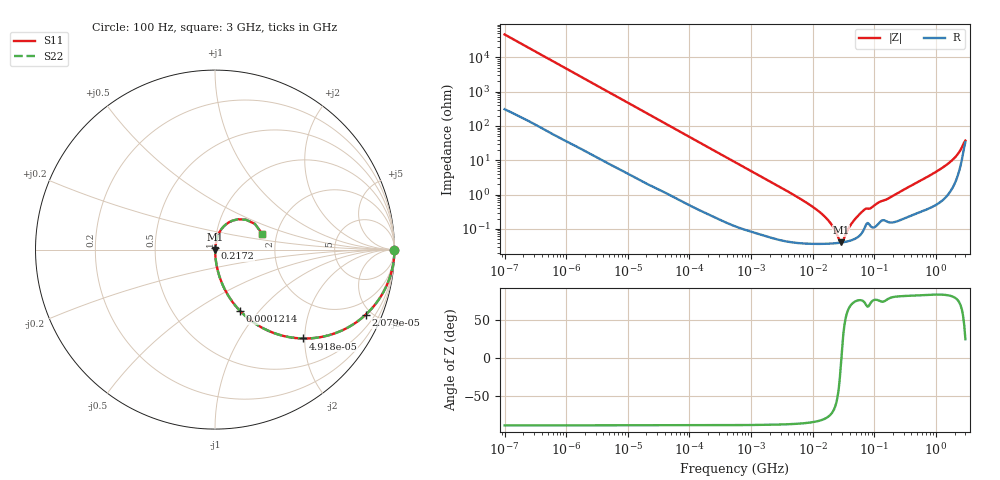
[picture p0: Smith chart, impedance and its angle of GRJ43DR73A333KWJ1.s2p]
!Murata Part Number: GRJ43DR73A333KWJ1
!These Parameters are Measured in Series Mode Connection
!Data Generated on Jun 19, 2026
!  o--ll--o
!Port1  Port2
!  o------o
!Operation Temp=25[degC], DC Bias Voltage=0[V]
!Freq. Start=100[Hz] Stop=3[GHz] 401[Steps]
# Hz S RI R 50
!Freq.(Hz) S11(Real) S11(Imag) S21(Real) S21(Imag) S12(Real) S12(Imag) S22(Real) S22(Imag)
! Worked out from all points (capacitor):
!   401 points, 100 Hz to 3 GHz, reference 50 ohm
!   read as one part in series: C = 34.1 nF near 109 Hz
!   lowest |Z| = 40.1 mohm at 28.73 MHz (marker M1)
!   series resonance near 29.17 MHz, so ESL is about 870 pH
!   S11 on the Smith chart (normalised r, x): 100 Hz: open; 20.79 kHz: 1.04, -4.61; 49.18 kHz: 1.02, -1.96; 121.4 kHz: 1.01, -0.80; 217.2 MHz: 1.00, +0.02; 3 GHz: 1.68, +0.31
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100  1 -0.00214  1.88e-05 0.00214  1.88e-05 0.00214  1 -0.00214
1788  0.9983 -0.0377  0.00172 0.0377  0.00172 0.0377  0.9983 -0.0377
6790  0.979 -0.1394  0.021 0.1394  0.021 0.1394  0.979 -0.1394
20793  0.8393 -0.3629  0.1607 0.3629  0.1607 0.3629  0.8393 -0.3629
31977  0.6912 -0.4574  0.3088 0.4574  0.3088 0.4574  0.6912 -0.4574
49177  0.4895 -0.4951  0.5105 0.4951  0.5105 0.4951  0.4895 -0.4951
121426  0.1397 -0.3416  0.8603 0.3416  0.8603 0.3416  0.1397 -0.3416
221826  0.0479 -0.208  0.9521 0.208  0.9521 0.208  0.0479 -0.208
547723  0.00905 -0.0883  0.9909 0.0883  0.9909 0.0883  0.00905 -0.0883
9794414  0.000386 -0.00449  0.9996 0.00449  0.9996 0.00449  0.000386 -0.00449
1.789277e7  0.000373 -0.00173  0.9996 0.00173  0.9996 0.00173  0.000373 -0.00173
2.635803e7  0.00039 -0.000347  0.9996 0.000347  0.9996 0.000347  0.00039 -0.000347
2.872754e7  0.000398 -5.2e-05  0.9996 5.2e-05  0.9996 5.2e-05  0.000398 -5.2e-05
3.131008e7  0.000408 0.000243  0.9996 -0.000243  0.9996 -0.000243  0.000408 0.000243
4.418008e7  0.00048 0.00148  0.9995 -0.00148  0.9995 -0.00148  0.00048 0.00148
6.508213e7  0.000852 0.00322  0.9991 -0.00322  0.9991 -0.00322  0.000852 0.00322
1.751444e8  0.00161 0.00786  0.9984 -0.00786  0.9984 -0.00786  0.00161 0.00786
2.172002e8  0.00169 0.00993  0.9983 -0.00993  0.9983 -0.00993  0.00169 0.00993
1.382454e9  0.012 0.0656  0.988 -0.0656  0.988 -0.0656  0.012 0.0656
2.219584e9  0.0497 0.1304  0.9503 -0.1304  0.9503 -0.1304  0.0497 0.1304
2.636591e9  0.1291 0.1691  0.8709 -0.1691  0.8709 -0.1691  0.1291 0.1691
3e9  0.2645 0.0858  0.7355 -0.0858  0.7355 -0.0858  0.2645 0.0858
